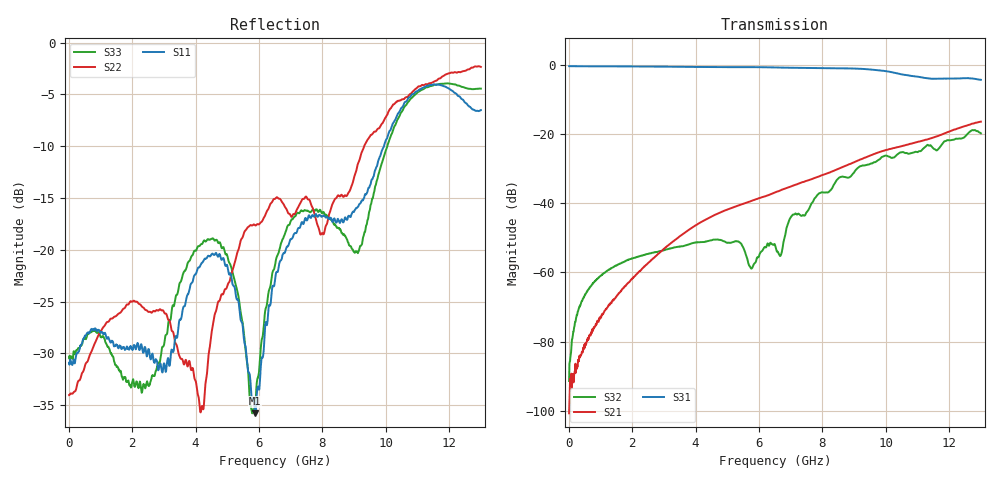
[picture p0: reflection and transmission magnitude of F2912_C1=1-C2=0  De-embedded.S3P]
! Integrated Device Technology
! Corporate Headquarters
! 6024 Silver Creek Valley Road
! San Jose, CA 95138  USA
! Phone:  1-408-284-8200
! Toll Free:  1-800-223-1366
! Webpage:  http://www.idt.com/
! Timing and RF Division
! 515 Groton Road, Suite 102
! Westford, MA 01886-6024
! Device:  F2912
! Description: High Reliability SP2T RF Switch
! Frequency:  9 kHz -  9 GHz
! Package:  4x4 mm QFN Plastic Package: 20 pin
! Ports:  3 RF, 5 DC
!  Pin  1  = GND
!  Pin  2  = GND
!  Pin  3  = RF1  =  Port 1
!  Pin  4  = GND
!  Pin  5  = GND
!  Pin  6  = GND
!  Pin  7  = GND
!  Pin  8  = RF_COM =  Port 3
!  Pin  9  = GND
!  Pin 10  = GND
!  Pin 11  = GND
!  Pin 12  = GND
!  Pin 13  = RF2  =  Port 2
!  Pin 14  = GND
!  Pin 15  = GND
!  Pin 16  = CTL2
!  Pin 17  = CTL1
!  Pin 18  = LogicCTL
!  Pin 19  = ModeCTL
!  Pin 20  = Vcc
! Logic:  3.3 V
! Mode:  2 pin control
! Voltage:  +3.30  Volts
! Current:  0.030 mA
! State:  RF1 Selected
! CTL1:  Logic HIGH
! CTL2:  Logic LOW
! Data:  The device was measured on a F2912 evaluation board which has
!  individual transmission lines to the RF pins.  Data was collected
!  using a calibrated network analyzer.  The evaluation board was
!  de-embedded using AFR (Keysight).
!  The reference plane is the edge of the package pin.
! Misc:  Action Tracker AT0438
! Date Measured:  2018-12-14
! Date:  2018-12-14  MJV
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# Hz S dB R 50
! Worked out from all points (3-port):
!   1300 points, 10 MHz to 13 GHz, reference 50 ohm
!   strongest paths, dB at 10 MHz, 3.26 GHz, 6.51 GHz, 9.76 GHz, 13 GHz:
!     S31: -0.3, -0.5, -0.7, -1.5, -4.2
!     S21: -100.8, -51.2, -36.9, -25.3, -16.4
!     S32: -91.4, -52.9, -52.1, -27.4, -19.7
!   lowest |S11| = -35.8 dB at 5.88 GHz (marker M1), VSWR 1.03, Z = 49 + j1.28 ohm
!   |S11| at or under -10 dB: start of sweep to 9.942 GHz
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1e7  -30.91 -1.8  -98.56 68.4  -0.31 -0.1
     -100.77 92.9  -34.02 178.8  -93.85 46.2
     -0.30 -0.1  -91.42 58.8  -30.30 -1.2
6.6e8  -27.91 34.0  -78.13 -121.5  -0.34 -5.5
       -77.96 -120.9  -30.17 146.1  -64.45 85.3
       -0.34 -5.5  -64.29 85.0  -27.95 30.3
1.85e9  -29.41 -6.7  -63.28 -145.1  -0.37 -15.2
        -63.20 -146.2  -25.28 176.2  -56.45 84.6
        -0.37 -15.3  -56.40 84.3  -32.70 -13.6
4.19e9  -21.28 71.0  -45.37 -172.5  -0.56 -35.2
        -45.35 -172.7  -35.18 172.4  -51.20 91.8
        -0.54 -35.3  -51.23 92.6  -19.43 12.3
4.53e9  -20.37 70.7  -43.74 -178.3  -0.58 -38.1
        -43.70 -178.6  -27.52 138.7  -50.79 91.6
        -0.57 -38.2  -50.62 91.3  -18.91 13.0
5.88e9  -35.76 126.5  -38.96 165.3  -0.60 -50.5
        -38.90 164.5  -17.64 169.6  -57.43 101.6
        -0.58 -50.5  -57.20 79.5  -35.28 -84.6
6.51e9  -22.82 174.7  -36.79 161.2  -0.68 -56.7
        -36.87 160.7  -15.08 -179.2  -53.60 -157.7
        -0.67 -56.8  -52.15 -141.3  -21.41 -124.4
8.92e9  -16.56 106.9  -28.35 146.2  -0.98 -84.3
        -28.41 140.9  -13.84 148.2  -31.15 -174.6
        -0.97 -84.3  -31.91 -178.1  -19.84 -111.7
1.157e10  -4.07 133.7  -20.63 85.6  -3.92 -114.5
          -20.70 84.5  -3.70 150.5  -23.53 122.6
          -3.95 -114.9  -24.48 127.2  -4.08 159.9
1.3e10  -6.52 98.3  -16.51 41.5  -4.25 -138.1
        -16.36 47.3  -2.35 127.2  -19.68 87.4
        -4.25 -138.2  -19.72 94.6  -4.45 149.1
